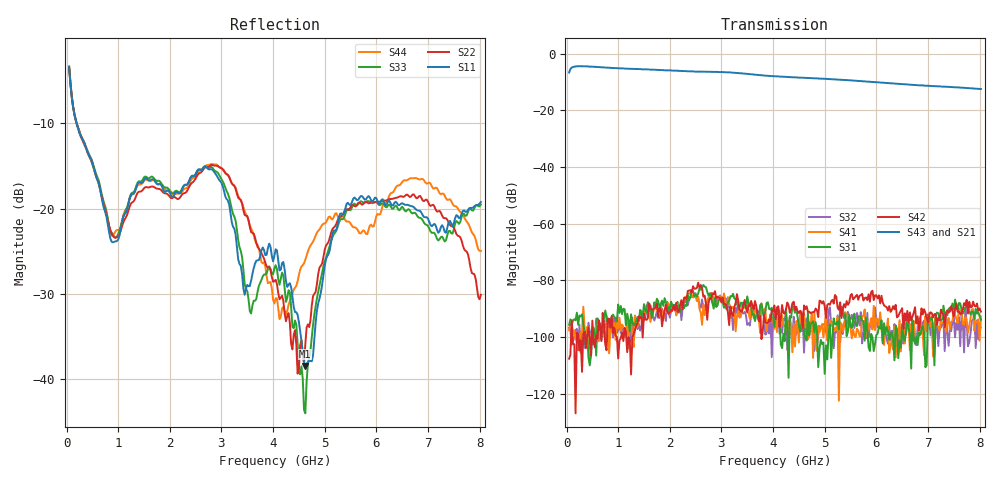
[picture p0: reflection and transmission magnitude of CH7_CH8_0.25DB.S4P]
!Agilent Technologies,E5071C,MY46316741,A.11.02
!Date: Mon Jun 01 10:30:40 2026
!Data & Calibration Information:
!1:CH7 INPUT 2:CH7 OUTPUT 3:CH8 INPUT 4:CH8 OUTPUT
!Freq	S11:SOLT4(ON)	S12:SOLT4(ON)	S13:SOLT4(ON)	S14:SOLT4(ON)
!	S21:SOLT4(ON)	S22:SOLT4(ON)	S23:SOLT4(ON)	S24:SOLT4(ON)
!	S31:SOLT4(ON)	S32:SOLT4(ON)	S33:SOLT4(ON)	S34:SOLT4(ON)
!	S41:SOLT4(ON)	S42:SOLT4(ON)	S43:SOLT4(ON)	S44:SOLT4(ON)
!PortZ  Port1:50+j0  Port2:50+j0  Port3:50+j0  Port4:50+j0
!Above PortZ is port z conversion or system Z0 setting when saving the data.
!When reading, reference impedance value at option line is always used.
# Hz S dB R 50
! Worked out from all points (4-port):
!   320 points, 50 MHz to 8.025 GHz, reference 50 ohm
!   strongest paths, dB at 50 MHz, 2.05 GHz, 4.05 GHz, 6.05 GHz, 8.025 GHz:
!     S43: -6.7, -6.0, -8.1, -10.2, -12.5
!     S21: -6.8, -6.1, -8.2, -10.4, -12.7
!     S42: -107.6, -90.8, -93.8, -85.3, -91.0
!     S31: -95.7, -88.8, -92.4, -96.5, -93.8
!     S41: -97.6, -89.5, -93.2, -96.3, -92.8
!     S32: -96.7, -88.5, -94.2, -94.0, -96.7
!   lowest |S11| = -38.5 dB at 4.625 GHz (marker M1), VSWR 1.02, Z = 51.1 + j0.541 ohm
!   |S11| at or under -10 dB: 197.2 MHz to end of sweep
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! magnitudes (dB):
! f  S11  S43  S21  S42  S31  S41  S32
! 50 MHz  -3.4  -6.7  -6.8  -107.6  -95.7  -97.6  -96.7
! 875 MHz  -23.9  -5.1  -5.1  -92.6  -92.8  -95.5  -96.5
! 2.925 GHz  -16.3  -6.5  -6.5  -85.7  -88.8  -87.9  -86.8
! 4.125 GHz  -27.3  -8.1  -8.3  -96.4  -94.0  -91.7  -98.9
! 4.625 GHz  -38.5  -8.6  -8.7  -90.1  -100.1  -96.5  -95.1
! 5.425 GHz  -19.4  -9.3  -9.5  -87.3  -99.7  -92.1  -96.1
! 8.025 GHz  -19.2  -12.5  -12.7  -91.0  -93.8  -92.8  -96.7
